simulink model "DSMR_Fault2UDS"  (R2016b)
settings: Solver=FixedStepDiscrete  StartTime=0.0  StopTime=10.0  FixedStep=0.02  RelTol=1e-3  EnableMultiTasking=on
undefined symbols (not defined in the file): bin2dec
libraries: simulink x312
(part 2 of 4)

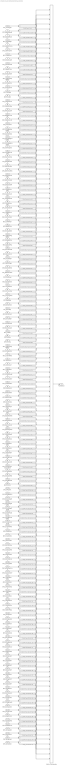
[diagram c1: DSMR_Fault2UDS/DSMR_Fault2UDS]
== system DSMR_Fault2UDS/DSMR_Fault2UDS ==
  DFC_CurrRngErr : Inport
  DFC_BattVoltRngErr : Inport  Port=2
  DFC_BattHVMsgTmt : Inport  Port=3
  DFC_BusHVMsgTmt : Inport  Port=4
  DFC_638LinCommErr : Inport  Port=5
  DFC_CellTempTmt : Inport  Port=6
  DFC_CellVoltTmt : Inport  Port=7
  DFC_InCanBusOff : Inport  Port=8
  DFC_VeCanBusOff : Inport  Port=9
  DFC_Msg2A3Tmt : Inport  Port=10
  DFC_RcMsg2A3Mis : Inport  Port=11
  DFC_ChkSumMsg2A3Err : Inport  Port=12
  DFC_RcMsg2A5Mis : Inport  Port=13
  DFC_RcMsg2A7Mis : Inport  Port=14
  DFC_CrashNpl : Inport  Port=15
  DFC_FuseNpl : Inport  Port=16
  DFC_Kl30cVoltLoErr : Inport  Port=17
  DFC_PosStuckMax : Inport  Port=18
  DFC_MPosStuckMin : Inport  Port=19
  DFC_MNegStuckMax : Inport  Port=20
  DFC_MNegStuckMin : Inport  Port=21
  DFC_PrStuckMin : Inport  Port=22
  DFC_DChrgPosStuckMax : Inport  Port=23
  DFC_DChrgPosStuckMin : Inport  Port=24
  DFC_DChrgNegStuckMax : Inport  Port=25
  DFC_DChrgNegStuckMin : Inport  Port=26
  DFC_HvPwrUpFail : Inport  Port=27
  DFC_DChrgPwrUpFail : Inport  Port=28
  DFC_BattTAlrmMax : Inport  Port=29
  DFC_BattTFaultMax : Inport  Port=30
  DFC_BattTAlrmMin : Inport  Port=31
  DFC_BattTFaultMin : Inport  Port=32
  DFC_BattTempVldMin : Inport  Port=33
  DFC_BattTCnstMax : Inport  Port=34
  DFC_BattTGradtMax : Inport  Port=35
  DFC_CellVoltAlrmMax : Inport  Port=36
  DFC_CellVoltFaultMax : Inport  Port=37
  DFC_CellVoltFusfMax : Inport  Port=38
  DFC_CellVoltAlrmMin : Inport  Port=39
  DFC_CellVoltFusfMin : Inport  Port=40
  DFC_CellVoltFaultMin : Inport  Port=41
  DFC_CellVoltVldMin : Inport  Port=42
  DFC_CellVoltNpl : Inport  Port=43
  DFC_Msg2E6Tmt : Inport  Port=44
  DFC_RcMsg2E6Mis : Inport  Port=45
  DFC_ChkSumMsg2E6Err : Inport  Port=46
  DFC_RcMsg2E1Mis : Inport  Port=47
  DFC_ChkSumMsg2E1Err : Inport  Port=48
  DFC_DcCanBusOff : Inport  Port=49
  DFC_DChrgTCnntMax : Inport  Port=50
  DFC_ChrgOCNpl : Inport  Port=51
  DFC_DisChOCNpl : Inport  Port=52
  DFC_BattVoltHiMax : Inport  Port=53
  DFC_BattVoltLoMin : Inport  Port=54
  DFC_ThmRnwy : Inport  Port=55
  DFC_AChrgPortOvrTemp : Inport  Port=56
  DFC_CurrOffsPlaus : Inport  Port=57
  DFC_CurrStukPlaus : Inport  Port=58
  DFC_CurrChrgPlaus : Inport  Port=59
  DFC_BattUNpl : Inport  Port=60
  DFC_BattVoltVld : Inport  Port=61
  DFC_PackUNpl : Inport  Port=62
  DFC_PackVoltVld : Inport  Port=63
  DFC_DChrgUNpl : Inport  Port=64
  DFC_DChrgVoltVld : Inport  Port=65
  DFC_BoardTempTmt : Inport  Port=66
  DFC_HvilMax : Inport  Port=67
  DFC_HvilMin : Inport  Port=68
  DFC_HvilSig : Inport  Port=69
  DFC_ChkSumMsg050Err : Inport  Port=70
  DFC_RcMsg050Mis : Inport  Port=71
  DFC_CrashHwNpl : Inport  Port=72
  DFC_IsoChkLv1 : Inport  Port=73
  DFC_IsoChkLv2 : Inport  Port=74
  DFC_InsResValdFault : Inport  Port=75
  DFC_Kl30OutRngErr : Inport  Port=76
  DFC_Kl30VoltLoErr : Inport  Port=77
  DFC_Kl30VoltHiErr : Inport  Port=78
  DFC_EepReadErr : Inport  Port=79
  DFC_BalStuckMax : Inport  Port=80
  DFC_BalStuckMin : Inport  Port=81
  DFC_CSCPwrSpyHiErr : Inport  Port=82
  DFC_CSCPwrSpyLoErr : Inport  Port=83
  DFC_CmcBordOTMax : Inport  Port=84
  DFC_BattTWarnMax : Inport  Port=85
  DFC_BattTWarnMin : Inport  Port=86
  DFC_BattTempVldMax : Inport  Port=87
  DFC_BattTHopMax : Inport  Port=88
  DFC_CellVoltRngHiErr : Inport  Port=89
  DFC_CellVoltRngLoErr : Inport  Port=90
  DFC_CellVoltWarnMax : Inport  Port=91
  DFC_CellVoltWarnMin : Inport  Port=92
  DFC_CellVoltVldMax : Inport  Port=93
  DFC_AChrgCurrMish : Inport  Port=94
  DFC_DChrgCurrMish : Inport  Port=95
  DFC_DChrgLowTempCurrMish : Inport  Port=96
  DFC_AChrgVoltMish : Inport  Port=97
  DFC_DChrgVoltMish : Inport  Port=98
  DFC_DChrgBattTMin : Inport  Port=99
  DFC_CC2Chk : Inport  Port=100
  DFC_APlusChk : Inport  Port=101
  DFC_DChrgMsgTmt : Inport  Port=102
  DFC_DChrgTNegElecMax : Inport  Port=103
  DFC_DChrgTNegElecMin : Inport  Port=104
  DFC_DChrgTNegElecSig : Inport  Port=105
  DFC_DChrgTPosElecMax : Inport  Port=106
  DFC_DChrgTPosElecMin : Inport  Port=107
  DFC_DChrgTPosElecSig : Inport  Port=108
  DFC_CcuSelfChkErr : Inport  Port=109
  DFC_ChrgOCMin : Inport  Port=110
  DFC_ChrgOCMax : Inport  Port=111
  DFC_DisChOCMin : Inport  Port=112
  DFC_DisChOCMax : Inport  Port=113
  DFC_SocRngLoMax : Inport  Port=114
  DFC_SocRngLoMin : Inport  Port=115
  DFC_SocRngHiMax : Inport  Port=116
  DFC_SocRngHiMin : Inport  Port=117
  DFC_InClntOverTmp : Inport  Port=118
  DFC_OutClntOverTmp : Inport  Port=119
  DFC_ClntDsTElecMax : Inport  Port=120
  DFC_ClntDsTElecMin : Inport  Port=121
  DFC_ClntDsTElecSig : Inport  Port=122
  DFC_ClntUsTElecMax : Inport  Port=123
  DFC_ClntUsTElecMin : Inport  Port=124
  DFC_ClntUsTElecSig : Inport  Port=125
  DFC_CoolPerfPlaus : Inport  Port=126
  DFC_HtgPerfPlaus : Inport  Port=127
  DFC_DChrgFobd : Inport  Port=128
  DFC_DChrgHvOnFail : Inport  Port=129
  DFC_AChgHVOnTmt : Inport  Port=130
  DFC_AChgHVOffTmt : Inport  Port=131
  DFC_AChgS2ClsdTmt : Inport  Port=132
  DFC_DChrgStakeErr : Inport  Port=133
  DFC_DChrgStkVoltErr : Inport  Port=134
  DFC_DChrgStkCurrErr : Inport  Port=135
  DFC_AChgPileRdyTmt : Inport  Port=136
  DFC_DChrgCHMTmt : Inport  Port=137
  DFC_DChrgCRMTmt : Inport  Port=138
  DFC_DChrgCMLTmt : Inport  Port=139
  DFC_DChrgCROTmt : Inport  Port=140
  DFC_DChrgCCSTmt : Inport  Port=141
  DFC_DChrgCSTTmt : Inport  Port=142
  DFC_DChrgCSDTmt : Inport  Port=143
  DFC_DChrgParaChk : Inport  Port=144
  DFC_DChrgCableChk : Inport  Port=145
  DFC_DChrgSLACTOut : Inport  Port=146
  DFC_DChrgCnntErr : Inport  Port=147
  DFC_DChrgLckErr : Inport  Port=148
  DFC_AChrgCnntErr : Inport  Port=149
  DFC_AChgLckTmt : Inport  Port=150
  DFC_AChgRdyPndiTmt : Inport  Port=151
  DFC_AChgRdyTmt : Inport  Port=152
  DFC_AChgingErr : Inport  Port=153
  DFC_AChgUnlckTmt : Inport  Port=154
  DFC_AChgFobd : Inport  Port=155
  DFC_SocValJmp : Inport  Port=156
  DSM_GetSFCErD : Subsystem  TreatAsAtomicUnit=on  RTWFcnName=TONV_10msTimeDebounce  RTWFileName=SrvLib
  DSM_GetSFCErD1 : Subsystem  TreatAsAtomicUnit=on  RTWFcnName=TONV_10msTimeDebounce  RTWFileName=SrvLib
  DSM_GetSFCErD10 : Subsystem  TreatAsAtomicUnit=on  RTWFcnName=TONV_10msTimeDebounce  RTWFileName=SrvLib
  DSM_GetSFCErD100 : Subsystem  TreatAsAtomicUnit=on  RTWFcnName=TONV_10msTimeDebounce  RTWFileName=SrvLib
  DSM_GetSFCErD101 : Subsystem  TreatAsAtomicUnit=on  RTWFcnName=TONV_10msTimeDebounce  RTWFileName=SrvLib
  DSM_GetSFCErD102 : Subsystem  TreatAsAtomicUnit=on  RTWFcnName=TONV_10msTimeDebounce  RTWFileName=SrvLib
  DSM_GetSFCErD103 : Subsystem  TreatAsAtomicUnit=on  RTWFcnName=TONV_10msTimeDebounce  RTWFileName=SrvLib
  DSM_GetSFCErD104 : Subsystem  TreatAsAtomicUnit=on  RTWFcnName=TONV_10msTimeDebounce  RTWFileName=SrvLib
  DSM_GetSFCErD105 : Subsystem  TreatAsAtomicUnit=on  RTWFcnName=TONV_10msTimeDebounce  RTWFileName=SrvLib
  DSM_GetSFCErD106 : Subsystem  TreatAsAtomicUnit=on  RTWFcnName=TONV_10msTimeDebounce  RTWFileName=SrvLib
  DSM_GetSFCErD107 : Subsystem  TreatAsAtomicUnit=on  RTWFcnName=TONV_10msTimeDebounce  RTWFileName=SrvLib
  DSM_GetSFCErD108 : Subsystem  TreatAsAtomicUnit=on  RTWFcnName=TONV_10msTimeDebounce  RTWFileName=SrvLib
  DSM_GetSFCErD109 : Subsystem  TreatAsAtomicUnit=on  RTWFcnName=TONV_10msTimeDebounce  RTWFileName=SrvLib
  DSM_GetSFCErD11 : Subsystem  TreatAsAtomicUnit=on  RTWFcnName=TONV_10msTimeDebounce  RTWFileName=SrvLib
  DSM_GetSFCErD110 : Subsystem  TreatAsAtomicUnit=on  RTWFcnName=TONV_10msTimeDebounce  RTWFileName=SrvLib
  DSM_GetSFCErD111 : Subsystem  TreatAsAtomicUnit=on  RTWFcnName=TONV_10msTimeDebounce  RTWFileName=SrvLib
  DSM_GetSFCErD112 : Subsystem  TreatAsAtomicUnit=on  RTWFcnName=TONV_10msTimeDebounce  RTWFileName=SrvLib
  DSM_GetSFCErD113 : Subsystem  TreatAsAtomicUnit=on  RTWFcnName=TONV_10msTimeDebounce  RTWFileName=SrvLib
  DSM_GetSFCErD114 : Subsystem  TreatAsAtomicUnit=on  RTWFcnName=TONV_10msTimeDebounce  RTWFileName=SrvLib
  DSM_GetSFCErD115 : Subsystem  TreatAsAtomicUnit=on  RTWFcnName=TONV_10msTimeDebounce  RTWFileName=SrvLib
  DSM_GetSFCErD116 : Subsystem  TreatAsAtomicUnit=on  RTWFcnName=TONV_10msTimeDebounce  RTWFileName=SrvLib
  DSM_GetSFCErD117 : Subsystem  TreatAsAtomicUnit=on  RTWFcnName=TONV_10msTimeDebounce  RTWFileName=SrvLib
  DSM_GetSFCErD118 : Subsystem  TreatAsAtomicUnit=on  RTWFcnName=TONV_10msTimeDebounce  RTWFileName=SrvLib
  DSM_GetSFCErD119 : Subsystem  TreatAsAtomicUnit=on  RTWFcnName=TONV_10msTimeDebounce  RTWFileName=SrvLib
  DSM_GetSFCErD12 : Subsystem  TreatAsAtomicUnit=on  RTWFcnName=TONV_10msTimeDebounce  RTWFileName=SrvLib
  DSM_GetSFCErD120 : Subsystem  TreatAsAtomicUnit=on  RTWFcnName=TONV_10msTimeDebounce  RTWFileName=SrvLib
  DSM_GetSFCErD121 : Subsystem  TreatAsAtomicUnit=on  RTWFcnName=TONV_10msTimeDebounce  RTWFileName=SrvLib
  DSM_GetSFCErD122 : Subsystem  TreatAsAtomicUnit=on  RTWFcnName=TONV_10msTimeDebounce  RTWFileName=SrvLib
  DSM_GetSFCErD123 : Subsystem  TreatAsAtomicUnit=on  RTWFcnName=TONV_10msTimeDebounce  RTWFileName=SrvLib
  DSM_GetSFCErD124 : Subsystem  TreatAsAtomicUnit=on  RTWFcnName=TONV_10msTimeDebounce  RTWFileName=SrvLib
  DSM_GetSFCErD125 : Subsystem  TreatAsAtomicUnit=on  RTWFcnName=TONV_10msTimeDebounce  RTWFileName=SrvLib
  DSM_GetSFCErD126 : Subsystem  TreatAsAtomicUnit=on  RTWFcnName=TONV_10msTimeDebounce  RTWFileName=SrvLib
  DSM_GetSFCErD127 : Subsystem  TreatAsAtomicUnit=on  RTWFcnName=TONV_10msTimeDebounce  RTWFileName=SrvLib
  DSM_GetSFCErD128 : Subsystem  TreatAsAtomicUnit=on  RTWFcnName=TONV_10msTimeDebounce  RTWFileName=SrvLib
  DSM_GetSFCErD129 : Subsystem  TreatAsAtomicUnit=on  RTWFcnName=TONV_10msTimeDebounce  RTWFileName=SrvLib
  DSM_GetSFCErD13 : Subsystem  TreatAsAtomicUnit=on  RTWFcnName=TONV_10msTimeDebounce  RTWFileName=SrvLib
  DSM_GetSFCErD130 : Subsystem  TreatAsAtomicUnit=on  RTWFcnName=TONV_10msTimeDebounce  RTWFileName=SrvLib
  DSM_GetSFCErD131 : Subsystem  TreatAsAtomicUnit=on  RTWFcnName=TONV_10msTimeDebounce  RTWFileName=SrvLib
  DSM_GetSFCErD132 : Subsystem  TreatAsAtomicUnit=on  RTWFcnName=TONV_10msTimeDebounce  RTWFileName=SrvLib
  DSM_GetSFCErD133 : Subsystem  TreatAsAtomicUnit=on  RTWFcnName=TONV_10msTimeDebounce  RTWFileName=SrvLib
  DSM_GetSFCErD134 : Subsystem  TreatAsAtomicUnit=on  RTWFcnName=TONV_10msTimeDebounce  RTWFileName=SrvLib
  DSM_GetSFCErD135 : Subsystem  TreatAsAtomicUnit=on  RTWFcnName=TONV_10msTimeDebounce  RTWFileName=SrvLib
  DSM_GetSFCErD136 : Subsystem  TreatAsAtomicUnit=on  RTWFcnName=TONV_10msTimeDebounce  RTWFileName=SrvLib
  DSM_GetSFCErD137 : Subsystem  TreatAsAtomicUnit=on  RTWFcnName=TONV_10msTimeDebounce  RTWFileName=SrvLib
  DSM_GetSFCErD138 : Subsystem  TreatAsAtomicUnit=on  RTWFcnName=TONV_10msTimeDebounce  RTWFileName=SrvLib
  DSM_GetSFCErD139 : Subsystem  TreatAsAtomicUnit=on  RTWFcnName=TONV_10msTimeDebounce  RTWFileName=SrvLib
  DSM_GetSFCErD14 : Subsystem  TreatAsAtomicUnit=on  RTWFcnName=TONV_10msTimeDebounce  RTWFileName=SrvLib
  DSM_GetSFCErD140 : Subsystem  TreatAsAtomicUnit=on  RTWFcnName=TONV_10msTimeDebounce  RTWFileName=SrvLib
  DSM_GetSFCErD141 : Subsystem  TreatAsAtomicUnit=on  RTWFcnName=TONV_10msTimeDebounce  RTWFileName=SrvLib
  DSM_GetSFCErD142 : Subsystem  TreatAsAtomicUnit=on  RTWFcnName=TONV_10msTimeDebounce  RTWFileName=SrvLib
  DSM_GetSFCErD143 : Subsystem  TreatAsAtomicUnit=on  RTWFcnName=TONV_10msTimeDebounce  RTWFileName=SrvLib
  DSM_GetSFCErD144 : Subsystem  TreatAsAtomicUnit=on  RTWFcnName=TONV_10msTimeDebounce  RTWFileName=SrvLib
  DSM_GetSFCErD145 : Subsystem  TreatAsAtomicUnit=on  RTWFcnName=TONV_10msTimeDebounce  RTWFileName=SrvLib
  DSM_GetSFCErD146 : Subsystem  TreatAsAtomicUnit=on  RTWFcnName=TONV_10msTimeDebounce  RTWFileName=SrvLib
  DSM_GetSFCErD147 : Subsystem  TreatAsAtomicUnit=on  RTWFcnName=TONV_10msTimeDebounce  RTWFileName=SrvLib
  DSM_GetSFCErD148 : Subsystem  TreatAsAtomicUnit=on  RTWFcnName=TONV_10msTimeDebounce  RTWFileName=SrvLib
  DSM_GetSFCErD149 : Subsystem  TreatAsAtomicUnit=on  RTWFcnName=TONV_10msTimeDebounce  RTWFileName=SrvLib
  DSM_GetSFCErD15 : Subsystem  TreatAsAtomicUnit=on  RTWFcnName=TONV_10msTimeDebounce  RTWFileName=SrvLib
  DSM_GetSFCErD150 : Subsystem  TreatAsAtomicUnit=on  RTWFcnName=TONV_10msTimeDebounce  RTWFileName=SrvLib
  DSM_GetSFCErD151 : Subsystem  TreatAsAtomicUnit=on  RTWFcnName=TONV_10msTimeDebounce  RTWFileName=SrvLib
  DSM_GetSFCErD152 : Subsystem  TreatAsAtomicUnit=on  RTWFcnName=TONV_10msTimeDebounce  RTWFileName=SrvLib
  DSM_GetSFCErD153 : Subsystem  TreatAsAtomicUnit=on  RTWFcnName=TONV_10msTimeDebounce  RTWFileName=SrvLib
  DSM_GetSFCErD154 : Subsystem  TreatAsAtomicUnit=on  RTWFcnName=TONV_10msTimeDebounce  RTWFileName=SrvLib
  DSM_GetSFCErD155 : Subsystem  TreatAsAtomicUnit=on  RTWFcnName=TONV_10msTimeDebounce  RTWFileName=SrvLib
  DSM_GetSFCErD16 : Subsystem  TreatAsAtomicUnit=on  RTWFcnName=TONV_10msTimeDebounce  RTWFileName=SrvLib
  DSM_GetSFCErD17 : Subsystem  TreatAsAtomicUnit=on  RTWFcnName=TONV_10msTimeDebounce  RTWFileName=SrvLib
  DSM_GetSFCErD18 : Subsystem  TreatAsAtomicUnit=on  RTWFcnName=TONV_10msTimeDebounce  RTWFileName=SrvLib
  DSM_GetSFCErD19 : Subsystem  TreatAsAtomicUnit=on  RTWFcnName=TONV_10msTimeDebounce  RTWFileName=SrvLib
  DSM_GetSFCErD2 : Subsystem  TreatAsAtomicUnit=on  RTWFcnName=TONV_10msTimeDebounce  RTWFileName=SrvLib
  DSM_GetSFCErD20 : Subsystem  TreatAsAtomicUnit=on  RTWFcnName=TONV_10msTimeDebounce  RTWFileName=SrvLib
  DSM_GetSFCErD21 : Subsystem  TreatAsAtomicUnit=on  RTWFcnName=TONV_10msTimeDebounce  RTWFileName=SrvLib
  DSM_GetSFCErD22 : Subsystem  TreatAsAtomicUnit=on  RTWFcnName=TONV_10msTimeDebounce  RTWFileName=SrvLib
  DSM_GetSFCErD23 : Subsystem  TreatAsAtomicUnit=on  RTWFcnName=TONV_10msTimeDebounce  RTWFileName=SrvLib
  DSM_GetSFCErD24 : Subsystem  TreatAsAtomicUnit=on  RTWFcnName=TONV_10msTimeDebounce  RTWFileName=SrvLib
  DSM_GetSFCErD25 : Subsystem  TreatAsAtomicUnit=on  RTWFcnName=TONV_10msTimeDebounce  RTWFileName=SrvLib
  DSM_GetSFCErD26 : Subsystem  TreatAsAtomicUnit=on  RTWFcnName=TONV_10msTimeDebounce  RTWFileName=SrvLib
  DSM_GetSFCErD27 : Subsystem  TreatAsAtomicUnit=on  RTWFcnName=TONV_10msTimeDebounce  RTWFileName=SrvLib
  DSM_GetSFCErD28 : Subsystem  TreatAsAtomicUnit=on  RTWFcnName=TONV_10msTimeDebounce  RTWFileName=SrvLib
  DSM_GetSFCErD29 : Subsystem  TreatAsAtomicUnit=on  RTWFcnName=TONV_10msTimeDebounce  RTWFileName=SrvLib
  DSM_GetSFCErD3 : Subsystem  TreatAsAtomicUnit=on  RTWFcnName=TONV_10msTimeDebounce  RTWFileName=SrvLib
  DSM_GetSFCErD30 : Subsystem  TreatAsAtomicUnit=on  RTWFcnName=TONV_10msTimeDebounce  RTWFileName=SrvLib
  DSM_GetSFCErD31 : Subsystem  TreatAsAtomicUnit=on  RTWFcnName=TONV_10msTimeDebounce  RTWFileName=SrvLib
  DSM_GetSFCErD32 : Subsystem  TreatAsAtomicUnit=on  RTWFcnName=TONV_10msTimeDebounce  RTWFileName=SrvLib
  DSM_GetSFCErD33 : Subsystem  TreatAsAtomicUnit=on  RTWFcnName=TONV_10msTimeDebounce  RTWFileName=SrvLib
  DSM_GetSFCErD34 : Subsystem  TreatAsAtomicUnit=on  RTWFcnName=TONV_10msTimeDebounce  RTWFileName=SrvLib
  DSM_GetSFCErD35 : Subsystem  TreatAsAtomicUnit=on  RTWFcnName=TONV_10msTimeDebounce  RTWFileName=SrvLib
  DSM_GetSFCErD36 : Subsystem  TreatAsAtomicUnit=on  RTWFcnName=TONV_10msTimeDebounce  RTWFileName=SrvLib
  DSM_GetSFCErD37 : Subsystem  TreatAsAtomicUnit=on  RTWFcnName=TONV_10msTimeDebounce  RTWFileName=SrvLib
  DSM_GetSFCErD38 : Subsystem  TreatAsAtomicUnit=on  RTWFcnName=TONV_10msTimeDebounce  RTWFileName=SrvLib
  DSM_GetSFCErD39 : Subsystem  TreatAsAtomicUnit=on  RTWFcnName=TONV_10msTimeDebounce  RTWFileName=SrvLib
  DSM_GetSFCErD4 : Subsystem  TreatAsAtomicUnit=on  RTWFcnName=TONV_10msTimeDebounce  RTWFileName=SrvLib
  DSM_GetSFCErD40 : Subsystem  TreatAsAtomicUnit=on  RTWFcnName=TONV_10msTimeDebounce  RTWFileName=SrvLib
  DSM_GetSFCErD41 : Subsystem  TreatAsAtomicUnit=on  RTWFcnName=TONV_10msTimeDebounce  RTWFileName=SrvLib
  DSM_GetSFCErD42 : Subsystem  TreatAsAtomicUnit=on  RTWFcnName=TONV_10msTimeDebounce  RTWFileName=SrvLib
  DSM_GetSFCErD43 : Subsystem  TreatAsAtomicUnit=on  RTWFcnName=TONV_10msTimeDebounce  RTWFileName=SrvLib
  DSM_GetSFCErD44 : Subsystem  TreatAsAtomicUnit=on  RTWFcnName=TONV_10msTimeDebounce  RTWFileName=SrvLib
  DSM_GetSFCErD45 : Subsystem  TreatAsAtomicUnit=on  RTWFcnName=TONV_10msTimeDebounce  RTWFileName=SrvLib
  DSM_GetSFCErD46 : Subsystem  TreatAsAtomicUnit=on  RTWFcnName=TONV_10msTimeDebounce  RTWFileName=SrvLib
  DSM_GetSFCErD47 : Subsystem  TreatAsAtomicUnit=on  RTWFcnName=TONV_10msTimeDebounce  RTWFileName=SrvLib
  DSM_GetSFCErD48 : Subsystem  TreatAsAtomicUnit=on  RTWFcnName=TONV_10msTimeDebounce  RTWFileName=SrvLib
  DSM_GetSFCErD49 : Subsystem  TreatAsAtomicUnit=on  RTWFcnName=TONV_10msTimeDebounce  RTWFileName=SrvLib
  DSM_GetSFCErD5 : Subsystem  TreatAsAtomicUnit=on  RTWFcnName=TONV_10msTimeDebounce  RTWFileName=SrvLib
  DSM_GetSFCErD50 : Subsystem  TreatAsAtomicUnit=on  RTWFcnName=TONV_10msTimeDebounce  RTWFileName=SrvLib
  DSM_GetSFCErD51 : Subsystem  TreatAsAtomicUnit=on  RTWFcnName=TONV_10msTimeDebounce  RTWFileName=SrvLib
  DSM_GetSFCErD52 : Subsystem  TreatAsAtomicUnit=on  RTWFcnName=TONV_10msTimeDebounce  RTWFileName=SrvLib
  DSM_GetSFCErD53 : Subsystem  TreatAsAtomicUnit=on  RTWFcnName=TONV_10msTimeDebounce  RTWFileName=SrvLib
  DSM_GetSFCErD54 : Subsystem  TreatAsAtomicUnit=on  RTWFcnName=TONV_10msTimeDebounce  RTWFileName=SrvLib
  DSM_GetSFCErD55 : Subsystem  TreatAsAtomicUnit=on  RTWFcnName=TONV_10msTimeDebounce  RTWFileName=SrvLib
  DSM_GetSFCErD56 : Subsystem  TreatAsAtomicUnit=on  RTWFcnName=TONV_10msTimeDebounce  RTWFileName=SrvLib
  DSM_GetSFCErD57 : Subsystem  TreatAsAtomicUnit=on  RTWFcnName=TONV_10msTimeDebounce  RTWFileName=SrvLib
  DSM_GetSFCErD58 : Subsystem  TreatAsAtomicUnit=on  RTWFcnName=TONV_10msTimeDebounce  RTWFileName=SrvLib
  DSM_GetSFCErD59 : Subsystem  TreatAsAtomicUnit=on  RTWFcnName=TONV_10msTimeDebounce  RTWFileName=SrvLib
  DSM_GetSFCErD6 : Subsystem  TreatAsAtomicUnit=on  RTWFcnName=TONV_10msTimeDebounce  RTWFileName=SrvLib
  DSM_GetSFCErD60 : Subsystem  TreatAsAtomicUnit=on  RTWFcnName=TONV_10msTimeDebounce  RTWFileName=SrvLib
  DSM_GetSFCErD61 : Subsystem  TreatAsAtomicUnit=on  RTWFcnName=TONV_10msTimeDebounce  RTWFileName=SrvLib
  DSM_GetSFCErD62 : Subsystem  TreatAsAtomicUnit=on  RTWFcnName=TONV_10msTimeDebounce  RTWFileName=SrvLib
  DSM_GetSFCErD63 : Subsystem  TreatAsAtomicUnit=on  RTWFcnName=TONV_10msTimeDebounce  RTWFileName=SrvLib
  DSM_GetSFCErD64 : Subsystem  TreatAsAtomicUnit=on  RTWFcnName=TONV_10msTimeDebounce  RTWFileName=SrvLib
  DSM_GetSFCErD65 : Subsystem  TreatAsAtomicUnit=on  RTWFcnName=TONV_10msTimeDebounce  RTWFileName=SrvLib
  DSM_GetSFCErD66 : Subsystem  TreatAsAtomicUnit=on  RTWFcnName=TONV_10msTimeDebounce  RTWFileName=SrvLib
  DSM_GetSFCErD67 : Subsystem  TreatAsAtomicUnit=on  RTWFcnName=TONV_10msTimeDebounce  RTWFileName=SrvLib
  DSM_GetSFCErD68 : Subsystem  TreatAsAtomicUnit=on  RTWFcnName=TONV_10msTimeDebounce  RTWFileName=SrvLib
  DSM_GetSFCErD69 : Subsystem  TreatAsAtomicUnit=on  RTWFcnName=TONV_10msTimeDebounce  RTWFileName=SrvLib
  DSM_GetSFCErD7 : Subsystem  TreatAsAtomicUnit=on  RTWFcnName=TONV_10msTimeDebounce  RTWFileName=SrvLib
  DSM_GetSFCErD70 : Subsystem  TreatAsAtomicUnit=on  RTWFcnName=TONV_10msTimeDebounce  RTWFileName=SrvLib
  DSM_GetSFCErD71 : Subsystem  TreatAsAtomicUnit=on  RTWFcnName=TONV_10msTimeDebounce  RTWFileName=SrvLib
  DSM_GetSFCErD72 : Subsystem  TreatAsAtomicUnit=on  RTWFcnName=TONV_10msTimeDebounce  RTWFileName=SrvLib
  DSM_GetSFCErD73 : Subsystem  TreatAsAtomicUnit=on  RTWFcnName=TONV_10msTimeDebounce  RTWFileName=SrvLib
  DSM_GetSFCErD74 : Subsystem  TreatAsAtomicUnit=on  RTWFcnName=TONV_10msTimeDebounce  RTWFileName=SrvLib
  DSM_GetSFCErD75 : Subsystem  TreatAsAtomicUnit=on  RTWFcnName=TONV_10msTimeDebounce  RTWFileName=SrvLib
  DSM_GetSFCErD76 : Subsystem  TreatAsAtomicUnit=on  RTWFcnName=TONV_10msTimeDebounce  RTWFileName=SrvLib
  DSM_GetSFCErD77 : Subsystem  TreatAsAtomicUnit=on  RTWFcnName=TONV_10msTimeDebounce  RTWFileName=SrvLib
  DSM_GetSFCErD78 : Subsystem  TreatAsAtomicUnit=on  RTWFcnName=TONV_10msTimeDebounce  RTWFileName=SrvLib
  DSM_GetSFCErD79 : Subsystem  TreatAsAtomicUnit=on  RTWFcnName=TONV_10msTimeDebounce  RTWFileName=SrvLib
  DSM_GetSFCErD8 : Subsystem  TreatAsAtomicUnit=on  RTWFcnName=TONV_10msTimeDebounce  RTWFileName=SrvLib
  DSM_GetSFCErD80 : Subsystem  TreatAsAtomicUnit=on  RTWFcnName=TONV_10msTimeDebounce  RTWFileName=SrvLib
  DSM_GetSFCErD81 : Subsystem  TreatAsAtomicUnit=on  RTWFcnName=TONV_10msTimeDebounce  RTWFileName=SrvLib
  DSM_GetSFCErD82 : Subsystem  TreatAsAtomicUnit=on  RTWFcnName=TONV_10msTimeDebounce  RTWFileName=SrvLib
  DSM_GetSFCErD83 : Subsystem  TreatAsAtomicUnit=on  RTWFcnName=TONV_10msTimeDebounce  RTWFileName=SrvLib
  DSM_GetSFCErD84 : Subsystem  TreatAsAtomicUnit=on  RTWFcnName=TONV_10msTimeDebounce  RTWFileName=SrvLib
  DSM_GetSFCErD85 : Subsystem  TreatAsAtomicUnit=on  RTWFcnName=TONV_10msTimeDebounce  RTWFileName=SrvLib
  DSM_GetSFCErD86 : Subsystem  TreatAsAtomicUnit=on  RTWFcnName=TONV_10msTimeDebounce  RTWFileName=SrvLib
  DSM_GetSFCErD87 : Subsystem  TreatAsAtomicUnit=on  RTWFcnName=TONV_10msTimeDebounce  RTWFileName=SrvLib
  DSM_GetSFCErD88 : Subsystem  TreatAsAtomicUnit=on  RTWFcnName=TONV_10msTimeDebounce  RTWFileName=SrvLib
  DSM_GetSFCErD89 : Subsystem  TreatAsAtomicUnit=on  RTWFcnName=TONV_10msTimeDebounce  RTWFileName=SrvLib
  DSM_GetSFCErD9 : Subsystem  TreatAsAtomicUnit=on  RTWFcnName=TONV_10msTimeDebounce  RTWFileName=SrvLib
  DSM_GetSFCErD90 : Subsystem  TreatAsAtomicUnit=on  RTWFcnName=TONV_10msTimeDebounce  RTWFileName=SrvLib
  DSM_GetSFCErD91 : Subsystem  TreatAsAtomicUnit=on  RTWFcnName=TONV_10msTimeDebounce  RTWFileName=SrvLib
  DSM_GetSFCErD92 : Subsystem  TreatAsAtomicUnit=on  RTWFcnName=TONV_10msTimeDebounce  RTWFileName=SrvLib
  DSM_GetSFCErD93 : Subsystem  TreatAsAtomicUnit=on  RTWFcnName=TONV_10msTimeDebounce  RTWFileName=SrvLib
  DSM_GetSFCErD94 : Subsystem  TreatAsAtomicUnit=on  RTWFcnName=TONV_10msTimeDebounce  RTWFileName=SrvLib
  DSM_GetSFCErD95 : Subsystem  TreatAsAtomicUnit=on  RTWFcnName=TONV_10msTimeDebounce  RTWFileName=SrvLib
  DSM_GetSFCErD96 : Subsystem  TreatAsAtomicUnit=on  RTWFcnName=TONV_10msTimeDebounce  RTWFileName=SrvLib
  DSM_GetSFCErD97 : Subsystem  TreatAsAtomicUnit=on  RTWFcnName=TONV_10msTimeDebounce  RTWFileName=SrvLib
  DSM_GetSFCErD98 : Subsystem  TreatAsAtomicUnit=on  RTWFcnName=TONV_10msTimeDebounce  RTWFileName=SrvLib
  DSM_GetSFCErD99 : Subsystem  TreatAsAtomicUnit=on  RTWFcnName=TONV_10msTimeDebounce  RTWFileName=SrvLib
  Vector Concatenate : Concatenate  NumInputs=156
  FaultStatus : Outport
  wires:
  DFC_CurrRngErr/1 -> DSM_GetSFCErD/1(DFC)
  DFC_BattVoltRngErr/1 -> DSM_GetSFCErD1/1(DFC)
  DFC_BattHVMsgTmt/1 -> DSM_GetSFCErD2/1(DFC)
  DFC_BusHVMsgTmt/1 -> DSM_GetSFCErD3/1(DFC)
  DFC_638LinCommErr/1 -> DSM_GetSFCErD4/1(DFC)
  DFC_CellTempTmt/1 -> DSM_GetSFCErD5/1(DFC)
  DFC_CellVoltTmt/1 -> DSM_GetSFCErD6/1(DFC)
  DFC_InCanBusOff/1 -> DSM_GetSFCErD7/1(DFC)
  DFC_VeCanBusOff/1 -> DSM_GetSFCErD8/1(DFC)
  DFC_Msg2A3Tmt/1 -> DSM_GetSFCErD9/1(DFC)
  DFC_RcMsg2A3Mis/1 -> DSM_GetSFCErD10/1(DFC)
  DFC_ChkSumMsg2A3Err/1 -> DSM_GetSFCErD11/1(DFC)
  DFC_RcMsg2A5Mis/1 -> DSM_GetSFCErD12/1(DFC)
  DFC_RcMsg2A7Mis/1 -> DSM_GetSFCErD13/1(DFC)
  DFC_CrashNpl/1 -> DSM_GetSFCErD14/1(DFC)
  DFC_FuseNpl/1 -> DSM_GetSFCErD15/1(DFC)
  DFC_Kl30cVoltLoErr/1 -> DSM_GetSFCErD16/1(DFC)
  DFC_PosStuckMax/1 -> DSM_GetSFCErD17/1(DFC)
  DFC_MPosStuckMin/1 -> DSM_GetSFCErD18/1(DFC)
  DFC_MNegStuckMax/1 -> DSM_GetSFCErD19/1(DFC)
  DFC_MNegStuckMin/1 -> DSM_GetSFCErD20/1(DFC)
  DFC_PrStuckMin/1 -> DSM_GetSFCErD21/1(DFC)
  DFC_DChrgPosStuckMax/1 -> DSM_GetSFCErD22/1(DFC)
  DFC_DChrgPosStuckMin/1 -> DSM_GetSFCErD23/1(DFC)
  DFC_DChrgNegStuckMax/1 -> DSM_GetSFCErD24/1(DFC)
  DFC_DChrgNegStuckMin/1 -> DSM_GetSFCErD25/1(DFC)
  DFC_HvPwrUpFail/1 -> DSM_GetSFCErD26/1(DFC)
  DFC_DChrgPwrUpFail/1 -> DSM_GetSFCErD27/1(DFC)
  DFC_BattTAlrmMax/1 -> DSM_GetSFCErD28/1(DFC)
  DFC_BattTFaultMax/1 -> DSM_GetSFCErD29/1(DFC)
  DFC_BattTAlrmMin/1 -> DSM_GetSFCErD30/1(DFC)
  DFC_BattTFaultMin/1 -> DSM_GetSFCErD31/1(DFC)
  DFC_BattTempVldMin/1 -> DSM_GetSFCErD32/1(DFC)
  DFC_BattTCnstMax/1 -> DSM_GetSFCErD33/1(DFC)
  DFC_BattTGradtMax/1 -> DSM_GetSFCErD34/1(DFC)
  DFC_CellVoltAlrmMax/1 -> DSM_GetSFCErD35/1(DFC)
  DFC_CellVoltFaultMax/1 -> DSM_GetSFCErD36/1(DFC)
  DFC_CellVoltFusfMax/1 -> DSM_GetSFCErD37/1(DFC)
  DFC_CellVoltAlrmMin/1 -> DSM_GetSFCErD38/1(DFC)
  DFC_CellVoltFusfMin/1 -> DSM_GetSFCErD39/1(DFC)
  DFC_CellVoltFaultMin/1 -> DSM_GetSFCErD40/1(DFC)
  DFC_CellVoltVldMin/1 -> DSM_GetSFCErD41/1(DFC)
  DFC_CellVoltNpl/1 -> DSM_GetSFCErD42/1(DFC)
  DFC_Msg2E6Tmt/1 -> DSM_GetSFCErD43/1(DFC)
  DFC_RcMsg2E6Mis/1 -> DSM_GetSFCErD44/1(DFC)
  DFC_ChkSumMsg2E6Err/1 -> DSM_GetSFCErD45/1(DFC)
  DFC_RcMsg2E1Mis/1 -> DSM_GetSFCErD46/1(DFC)
  DFC_ChkSumMsg2E1Err/1 -> DSM_GetSFCErD47/1(DFC)
  DFC_DcCanBusOff/1 -> DSM_GetSFCErD48/1(DFC)
  DFC_DChrgTCnntMax/1 -> DSM_GetSFCErD49/1(DFC)
  DFC_ChrgOCNpl/1 -> DSM_GetSFCErD50/1(DFC)
  DFC_DisChOCNpl/1 -> DSM_GetSFCErD51/1(DFC)
  DFC_BattVoltHiMax/1 -> DSM_GetSFCErD52/1(DFC)
  DFC_BattVoltLoMin/1 -> DSM_GetSFCErD53/1(DFC)
  DFC_ThmRnwy/1 -> DSM_GetSFCErD54/1(DFC)
  DFC_AChrgPortOvrTemp/1 -> DSM_GetSFCErD55/1(DFC)
  DFC_CurrOffsPlaus/1 -> DSM_GetSFCErD56/1(DFC)
  DFC_CurrStukPlaus/1 -> DSM_GetSFCErD57/1(DFC)
  DFC_CurrChrgPlaus/1 -> DSM_GetSFCErD58/1(DFC)
  DFC_BattUNpl/1 -> DSM_GetSFCErD59/1(DFC)
  DFC_BattVoltVld/1 -> DSM_GetSFCErD60/1(DFC)
  DFC_PackUNpl/1 -> DSM_GetSFCErD61/1(DFC)
  DFC_PackVoltVld/1 -> DSM_GetSFCErD62/1(DFC)
  DFC_DChrgUNpl/1 -> DSM_GetSFCErD63/1(DFC)
  DFC_DChrgVoltVld/1 -> DSM_GetSFCErD64/1(DFC)
  DFC_BoardTempTmt/1 -> DSM_GetSFCErD65/1(DFC)
  DFC_HvilMax/1 -> DSM_GetSFCErD66/1(DFC)
  DFC_HvilMin/1 -> DSM_GetSFCErD67/1(DFC)
  DFC_HvilSig/1 -> DSM_GetSFCErD68/1(DFC)
  DFC_ChkSumMsg050Err/1 -> DSM_GetSFCErD69/1(DFC)
  DFC_RcMsg050Mis/1 -> DSM_GetSFCErD70/1(DFC)
  DFC_CrashHwNpl/1 -> DSM_GetSFCErD71/1(DFC)
  DFC_IsoChkLv1/1 -> DSM_GetSFCErD72/1(DFC)
  DFC_IsoChkLv2/1 -> DSM_GetSFCErD73/1(DFC)
  DFC_InsResValdFault/1 -> DSM_GetSFCErD74/1(DFC)
  DFC_Kl30OutRngErr/1 -> DSM_GetSFCErD75/1(DFC)
  DFC_Kl30VoltLoErr/1 -> DSM_GetSFCErD76/1(DFC)
  DFC_Kl30VoltHiErr/1 -> DSM_GetSFCErD77/1(DFC)
  DFC_EepReadErr/1 -> DSM_GetSFCErD78/1(DFC)
  DFC_BalStuckMax/1 -> DSM_GetSFCErD79/1(DFC)
  DFC_BalStuckMin/1 -> DSM_GetSFCErD80/1(DFC)
  DFC_CSCPwrSpyHiErr/1 -> DSM_GetSFCErD81/1(DFC)
  DFC_CSCPwrSpyLoErr/1 -> DSM_GetSFCErD82/1(DFC)
  DFC_CmcBordOTMax/1 -> DSM_GetSFCErD83/1(DFC)
  DFC_BattTWarnMax/1 -> DSM_GetSFCErD84/1(DFC)
  DFC_BattTWarnMin/1 -> DSM_GetSFCErD85/1(DFC)
  DFC_BattTempVldMax/1 -> DSM_GetSFCErD86/1(DFC)
  DFC_BattTHopMax/1 -> DSM_GetSFCErD87/1(DFC)
  DFC_CellVoltRngHiErr/1 -> DSM_GetSFCErD88/1(DFC)
  DFC_CellVoltRngLoErr/1 -> DSM_GetSFCErD89/1(DFC)
  DFC_CellVoltWarnMax/1 -> DSM_GetSFCErD90/1(DFC)
  DFC_CellVoltWarnMin/1 -> DSM_GetSFCErD91/1(DFC)
  DFC_CellVoltVldMax/1 -> DSM_GetSFCErD92/1(DFC)
  DFC_AChrgCurrMish/1 -> DSM_GetSFCErD93/1(DFC)
  DFC_DChrgCurrMish/1 -> DSM_GetSFCErD94/1(DFC)
  DFC_DChrgLowTempCurrMish/1 -> DSM_GetSFCErD95/1(DFC)
  DFC_AChrgVoltMish/1 -> DSM_GetSFCErD96/1(DFC)
  DFC_DChrgVoltMish/1 -> DSM_GetSFCErD97/1(DFC)
  DFC_DChrgBattTMin/1 -> DSM_GetSFCErD98/1(DFC)
  DFC_CC2Chk/1 -> DSM_GetSFCErD99/1(DFC)
  DFC_APlusChk/1 -> DSM_GetSFCErD100/1(DFC)
  DFC_DChrgMsgTmt/1 -> DSM_GetSFCErD101/1(DFC)
  DFC_DChrgTNegElecMax/1 -> DSM_GetSFCErD102/1(DFC)
  DFC_DChrgTNegElecMin/1 -> DSM_GetSFCErD103/1(DFC)
  DFC_DChrgTNegElecSig/1 -> DSM_GetSFCErD104/1(DFC)
  DFC_DChrgTPosElecMax/1 -> DSM_GetSFCErD105/1(DFC)
  DFC_DChrgTPosElecMin/1 -> DSM_GetSFCErD106/1(DFC)
  DFC_DChrgTPosElecSig/1 -> DSM_GetSFCErD107/1(DFC)
  DFC_CcuSelfChkErr/1 -> DSM_GetSFCErD108/1(DFC)
  DFC_ChrgOCMax/1 -> DSM_GetSFCErD119/1(DFC)
  DFC_DisChOCMin/1 -> DSM_GetSFCErD120/1(DFC)
  DFC_DisChOCMax/1 -> DSM_GetSFCErD121/1(DFC)
  DFC_SocRngLoMax/1 -> DSM_GetSFCErD122/1(DFC)
  DFC_SocRngLoMin/1 -> DSM_GetSFCErD123/1(DFC)
  DFC_SocRngHiMax/1 -> DSM_GetSFCErD124/1(DFC)
  DFC_SocRngHiMin/1 -> DSM_GetSFCErD125/1(DFC)
  DFC_InClntOverTmp/1 -> DSM_GetSFCErD126/1(DFC)
  DFC_OutClntOverTmp/1 -> DSM_GetSFCErD127/1(DFC)
  DFC_ClntDsTElecMax/1 -> DSM_GetSFCErD128/1(DFC)
  DFC_ClntDsTElecMin/1 -> DSM_GetSFCErD129/1(DFC)
  DFC_ClntDsTElecSig/1 -> DSM_GetSFCErD130/1(DFC)
  DFC_ClntUsTElecMax/1 -> DSM_GetSFCErD131/1(DFC)
  DFC_ClntUsTElecMin/1 -> DSM_GetSFCErD132/1(DFC)
  DFC_ClntUsTElecSig/1 -> DSM_GetSFCErD133/1(DFC)
  DFC_CoolPerfPlaus/1 -> DSM_GetSFCErD134/1(DFC)
  DFC_HtgPerfPlaus/1 -> DSM_GetSFCErD135/1(DFC)
  DFC_DChrgFobd/1 -> DSM_GetSFCErD136/1(DFC)
  DFC_DChrgHvOnFail/1 -> DSM_GetSFCErD137/1(DFC)
  DFC_AChgHVOnTmt/1 -> DSM_GetSFCErD138/1(DFC)
  DFC_AChgHVOffTmt/1 -> DSM_GetSFCErD139/1(DFC)
  DFC_AChgS2ClsdTmt/1 -> DSM_GetSFCErD140/1(DFC)
  DFC_DChrgStakeErr/1 -> DSM_GetSFCErD109/1(DFC)
  DFC_DChrgStkVoltErr/1 -> DSM_GetSFCErD110/1(DFC)
  DFC_DChrgStkCurrErr/1 -> DSM_GetSFCErD111/1(DFC)
  DFC_AChgPileRdyTmt/1 -> DSM_GetSFCErD112/1(DFC)
  DFC_DChrgCHMTmt/1 -> DSM_GetSFCErD113/1(DFC)
  DFC_DChrgCRMTmt/1 -> DSM_GetSFCErD114/1(DFC)
  DFC_DChrgCMLTmt/1 -> DSM_GetSFCErD115/1(DFC)
  DFC_DChrgCROTmt/1 -> DSM_GetSFCErD116/1(DFC)
  DFC_DChrgCCSTmt/1 -> DSM_GetSFCErD117/1(DFC)
  DFC_ChrgOCMin/1 -> DSM_GetSFCErD118/1(DFC)
  DFC_DChrgCSTTmt/1 -> DSM_GetSFCErD141/1(DFC)
  DFC_DChrgCSDTmt/1 -> DSM_GetSFCErD142/1(DFC)
  DFC_DChrgParaChk/1 -> DSM_GetSFCErD143/1(DFC)
  DFC_DChrgCableChk/1 -> DSM_GetSFCErD144/1(DFC)
  DFC_DChrgSLACTOut/1 -> DSM_GetSFCErD145/1(DFC)
  DFC_DChrgCnntErr/1 -> DSM_GetSFCErD146/1(DFC)
  DFC_DChrgLckErr/1 -> DSM_GetSFCErD147/1(DFC)
  DFC_AChrgCnntErr/1 -> DSM_GetSFCErD148/1(DFC)
  DFC_AChgLckTmt/1 -> DSM_GetSFCErD149/1(DFC)
  DFC_AChgRdyPndiTmt/1 -> DSM_GetSFCErD150/1(DFC)
  DFC_AChgRdyTmt/1 -> DSM_GetSFCErD151/1(DFC)
  DFC_AChgingErr/1 -> DSM_GetSFCErD152/1(DFC)
  DFC_AChgUnlckTmt/1 -> DSM_GetSFCErD153/1(DFC)
  DFC_AChgFobd/1 -> DSM_GetSFCErD154/1(DFC)
  DFC_SocValJmp/1 -> DSM_GetSFCErD155/1(DFC)
  DSM_GetSFCErD/1(y) -> Vector Concatenate/1
  DSM_GetSFCErD1/1(y) -> Vector Concatenate/2
  DSM_GetSFCErD2/1(y) -> Vector Concatenate/3
  DSM_GetSFCErD3/1(y) -> Vector Concatenate/4
  DSM_GetSFCErD4/1(y) -> Vector Concatenate/5
  DSM_GetSFCErD5/1(y) -> Vector Concatenate/6
  DSM_GetSFCErD6/1(y) -> Vector Concatenate/7
  DSM_GetSFCErD7/1(y) -> Vector Concatenate/8
  DSM_GetSFCErD8/1(y) -> Vector Concatenate/9
  DSM_GetSFCErD9/1(y) -> Vector Concatenate/10
  DSM_GetSFCErD10/1(y) -> Vector Concatenate/11
  DSM_GetSFCErD11/1(y) -> Vector Concatenate/12
  DSM_GetSFCErD12/1(y) -> Vector Concatenate/13
  DSM_GetSFCErD13/1(y) -> Vector Concatenate/14
  DSM_GetSFCErD14/1(y) -> Vector Concatenate/15
  DSM_GetSFCErD15/1(y) -> Vector Concatenate/16
  DSM_GetSFCErD16/1(y) -> Vector Concatenate/17
  DSM_GetSFCErD17/1(y) -> Vector Concatenate/18
  DSM_GetSFCErD18/1(y) -> Vector Concatenate/19
  DSM_GetSFCErD19/1(y) -> Vector Concatenate/20
  DSM_GetSFCErD20/1(y) -> Vector Concatenate/21
  DSM_GetSFCErD21/1(y) -> Vector Concatenate/22
  DSM_GetSFCErD22/1(y) -> Vector Concatenate/23
  DSM_GetSFCErD23/1(y) -> Vector Concatenate/24
  DSM_GetSFCErD24/1(y) -> Vector Concatenate/25
  DSM_GetSFCErD25/1(y) -> Vector Concatenate/26
  DSM_GetSFCErD26/1(y) -> Vector Concatenate/27
  DSM_GetSFCErD27/1(y) -> Vector Concatenate/28
  DSM_GetSFCErD28/1(y) -> Vector Concatenate/29
  DSM_GetSFCErD29/1(y) -> Vector Concatenate/30
  DSM_GetSFCErD30/1(y) -> Vector Concatenate/31
  DSM_GetSFCErD31/1(y) -> Vector Concatenate/32
  DSM_GetSFCErD32/1(y) -> Vector Concatenate/33
  DSM_GetSFCErD33/1(y) -> Vector Concatenate/34
  DSM_GetSFCErD34/1(y) -> Vector Concatenate/35
  DSM_GetSFCErD35/1(y) -> Vector Concatenate/36
  DSM_GetSFCErD36/1(y) -> Vector Concatenate/37
  DSM_GetSFCErD37/1(y) -> Vector Concatenate/38
  DSM_GetSFCErD38/1(y) -> Vector Concatenate/39
  DSM_GetSFCErD39/1(y) -> Vector Concatenate/40
  DSM_GetSFCErD40/1(y) -> Vector Concatenate/41
  DSM_GetSFCErD41/1(y) -> Vector Concatenate/42
  DSM_GetSFCErD42/1(y) -> Vector Concatenate/43
  DSM_GetSFCErD43/1(y) -> Vector Concatenate/44
  DSM_GetSFCErD44/1(y) -> Vector Concatenate/45
  DSM_GetSFCErD45/1(y) -> Vector Concatenate/46
  DSM_GetSFCErD46/1(y) -> Vector Concatenate/47
  DSM_GetSFCErD47/1(y) -> Vector Concatenate/48
  DSM_GetSFCErD48/1(y) -> Vector Concatenate/49
  DSM_GetSFCErD49/1(y) -> Vector Concatenate/50
  DSM_GetSFCErD50/1(y) -> Vector Concatenate/51
  DSM_GetSFCErD51/1(y) -> Vector Concatenate/52
  DSM_GetSFCErD52/1(y) -> Vector Concatenate/53
  DSM_GetSFCErD53/1(y) -> Vector Concatenate/54
  DSM_GetSFCErD54/1(y) -> Vector Concatenate/55
  DSM_GetSFCErD55/1(y) -> Vector Concatenate/56
  DSM_GetSFCErD56/1(y) -> Vector Concatenate/57
  DSM_GetSFCErD57/1(y) -> Vector Concatenate/58
  DSM_GetSFCErD58/1(y) -> Vector Concatenate/59
  DSM_GetSFCErD59/1(y) -> Vector Concatenate/60
  DSM_GetSFCErD60/1(y) -> Vector Concatenate/61
  DSM_GetSFCErD61/1(y) -> Vector Concatenate/62
  DSM_GetSFCErD62/1(y) -> Vector Concatenate/63
  DSM_GetSFCErD63/1(y) -> Vector Concatenate/64
  DSM_GetSFCErD64/1(y) -> Vector Concatenate/65
  DSM_GetSFCErD65/1(y) -> Vector Concatenate/66
  DSM_GetSFCErD66/1(y) -> Vector Concatenate/67
  DSM_GetSFCErD67/1(y) -> Vector Concatenate/68
  DSM_GetSFCErD68/1(y) -> Vector Concatenate/69
  DSM_GetSFCErD69/1(y) -> Vector Concatenate/70
  DSM_GetSFCErD70/1(y) -> Vector Concatenate/71
  DSM_GetSFCErD71/1(y) -> Vector Concatenate/72
  DSM_GetSFCErD72/1(y) -> Vector Concatenate/73
  DSM_GetSFCErD73/1(y) -> Vector Concatenate/74
  DSM_GetSFCErD74/1(y) -> Vector Concatenate/75
  DSM_GetSFCErD75/1(y) -> Vector Concatenate/76
  DSM_GetSFCErD76/1(y) -> Vector Concatenate/77
  DSM_GetSFCErD77/1(y) -> Vector Concatenate/78
  DSM_GetSFCErD78/1(y) -> Vector Concatenate/79
  DSM_GetSFCErD79/1(y) -> Vector Concatenate/80
  DSM_GetSFCErD80/1(y) -> Vector Concatenate/81
  DSM_GetSFCErD81/1(y) -> Vector Concatenate/82
  DSM_GetSFCErD82/1(y) -> Vector Concatenate/83
  DSM_GetSFCErD83/1(y) -> Vector Concatenate/84
  DSM_GetSFCErD84/1(y) -> Vector Concatenate/85
  DSM_GetSFCErD85/1(y) -> Vector Concatenate/86
  DSM_GetSFCErD86/1(y) -> Vector Concatenate/87
  DSM_GetSFCErD87/1(y) -> Vector Concatenate/88
  DSM_GetSFCErD88/1(y) -> Vector Concatenate/89
  DSM_GetSFCErD89/1(y) -> Vector Concatenate/90
  DSM_GetSFCErD90/1(y) -> Vector Concatenate/91
  DSM_GetSFCErD91/1(y) -> Vector Concatenate/92
  DSM_GetSFCErD92/1(y) -> Vector Concatenate/93
  DSM_GetSFCErD93/1(y) -> Vector Concatenate/94
  DSM_GetSFCErD94/1(y) -> Vector Concatenate/95
  DSM_GetSFCErD95/1(y) -> Vector Concatenate/96
  DSM_GetSFCErD96/1(y) -> Vector Concatenate/97
  DSM_GetSFCErD97/1(y) -> Vector Concatenate/98
  DSM_GetSFCErD98/1(y) -> Vector Concatenate/99
  DSM_GetSFCErD99/1(y) -> Vector Concatenate/100
  DSM_GetSFCErD100/1(y) -> Vector Concatenate/101
  DSM_GetSFCErD101/1(y) -> Vector Concatenate/102
  DSM_GetSFCErD102/1(y) -> Vector Concatenate/103
  DSM_GetSFCErD103/1(y) -> Vector Concatenate/104
  DSM_GetSFCErD104/1(y) -> Vector Concatenate/105
  DSM_GetSFCErD105/1(y) -> Vector Concatenate/106
  DSM_GetSFCErD106/1(y) -> Vector Concatenate/107
  DSM_GetSFCErD107/1(y) -> Vector Concatenate/108
  DSM_GetSFCErD108/1(y) -> Vector Concatenate/109
  DSM_GetSFCErD118/1(y) -> Vector Concatenate/110
  DSM_GetSFCErD119/1(y) -> Vector Concatenate/111
  DSM_GetSFCErD120/1(y) -> Vector Concatenate/112
  DSM_GetSFCErD121/1(y) -> Vector Concatenate/113
  DSM_GetSFCErD122/1(y) -> Vector Concatenate/114
  DSM_GetSFCErD123/1(y) -> Vector Concatenate/115
  DSM_GetSFCErD124/1(y) -> Vector Concatenate/116
  DSM_GetSFCErD125/1(y) -> Vector Concatenate/117
  DSM_GetSFCErD126/1(y) -> Vector Concatenate/118
  DSM_GetSFCErD127/1(y) -> Vector Concatenate/119
  DSM_GetSFCErD128/1(y) -> Vector Concatenate/120
  DSM_GetSFCErD129/1(y) -> Vector Concatenate/121
  DSM_GetSFCErD130/1(y) -> Vector Concatenate/122
  DSM_GetSFCErD131/1(y) -> Vector Concatenate/123
  DSM_GetSFCErD132/1(y) -> Vector Concatenate/124
  DSM_GetSFCErD133/1(y) -> Vector Concatenate/125
  DSM_GetSFCErD134/1(y) -> Vector Concatenate/126
  DSM_GetSFCErD135/1(y) -> Vector Concatenate/127
  DSM_GetSFCErD136/1(y) -> Vector Concatenate/128
  DSM_GetSFCErD137/1(y) -> Vector Concatenate/129
  DSM_GetSFCErD138/1(y) -> Vector Concatenate/130
  DSM_GetSFCErD139/1(y) -> Vector Concatenate/131
  DSM_GetSFCErD140/1(y) -> Vector Concatenate/132
  DSM_GetSFCErD109/1(y) -> Vector Concatenate/133
  DSM_GetSFCErD110/1(y) -> Vector Concatenate/134
  DSM_GetSFCErD111/1(y) -> Vector Concatenate/135
  DSM_GetSFCErD112/1(y) -> Vector Concatenate/136
  DSM_GetSFCErD113/1(y) -> Vector Concatenate/137
  DSM_GetSFCErD114/1(y) -> Vector Concatenate/138
  DSM_GetSFCErD115/1(y) -> Vector Concatenate/139
  DSM_GetSFCErD116/1(y) -> Vector Concatenate/140
  DSM_GetSFCErD117/1(y) -> Vector Concatenate/141
  DSM_GetSFCErD141/1(y) -> Vector Concatenate/142
  DSM_GetSFCErD142/1(y) -> Vector Concatenate/143
  DSM_GetSFCErD143/1(y) -> Vector Concatenate/144
  DSM_GetSFCErD144/1(y) -> Vector Concatenate/145
  DSM_GetSFCErD145/1(y) -> Vector Concatenate/146
  DSM_GetSFCErD146/1(y) -> Vector Concatenate/147
  DSM_GetSFCErD147/1(y) -> Vector Concatenate/148
  DSM_GetSFCErD148/1(y) -> Vector Concatenate/149
  DSM_GetSFCErD149/1(y) -> Vector Concatenate/150
  DSM_GetSFCErD150/1(y) -> Vector Concatenate/151
  DSM_GetSFCErD151/1(y) -> Vector Concatenate/152
  DSM_GetSFCErD152/1(y) -> Vector Concatenate/153
  DSM_GetSFCErD153/1(y) -> Vector Concatenate/154
  DSM_GetSFCErD154/1(y) -> Vector Concatenate/155
  DSM_GetSFCErD155/1(y) -> Vector Concatenate/156
  Vector Concatenate/1 -> FaultStatus/1

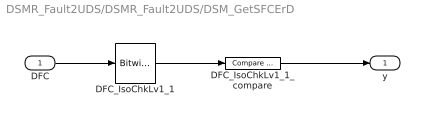
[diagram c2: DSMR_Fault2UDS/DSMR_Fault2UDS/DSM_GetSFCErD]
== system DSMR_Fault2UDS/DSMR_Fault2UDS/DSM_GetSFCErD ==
  DFC : Inport  OutDataTypeStr=uint8
  DFC_IsoChkLv1_1 : simulink/Logic and Bit Operations/Bitwise Operator  logicop=AND  UseBitMask=on  BitMask=bin2dec('00011000')  BitMaskRealWorld=Stored Integer
  DFC_IsoChkLv1_1_compare : simulink/Logic and Bit Operations/Compare To Constant  relop===  const=24  OutDataTypeStr=boolean
  y : Outport
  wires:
  DFC_IsoChkLv1_1_compare/1 -> y/1
  DFC/1 -> DFC_IsoChkLv1_1/1
  DFC_IsoChkLv1_1/1 -> DFC_IsoChkLv1_1_compare/1

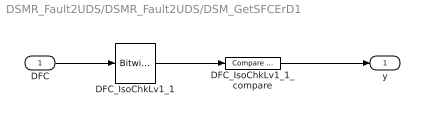
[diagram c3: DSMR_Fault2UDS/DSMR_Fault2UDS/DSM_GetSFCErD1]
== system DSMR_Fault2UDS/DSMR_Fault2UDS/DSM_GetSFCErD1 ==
  DFC : Inport  OutDataTypeStr=uint8
  DFC_IsoChkLv1_1 : simulink/Logic and Bit Operations/Bitwise Operator  logicop=AND  UseBitMask=on  BitMask=bin2dec('00011000')  BitMaskRealWorld=Stored Integer
  DFC_IsoChkLv1_1_compare : simulink/Logic and Bit Operations/Compare To Constant  relop===  const=24  OutDataTypeStr=boolean
  y : Outport
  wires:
  DFC_IsoChkLv1_1_compare/1 -> y/1
  DFC/1 -> DFC_IsoChkLv1_1/1
  DFC_IsoChkLv1_1/1 -> DFC_IsoChkLv1_1_compare/1

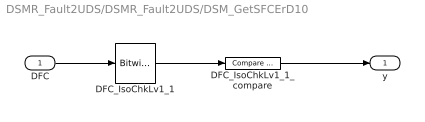
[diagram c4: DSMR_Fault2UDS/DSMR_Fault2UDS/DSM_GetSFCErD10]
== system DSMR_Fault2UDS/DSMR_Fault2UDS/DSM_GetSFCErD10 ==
  DFC : Inport  OutDataTypeStr=uint8
  DFC_IsoChkLv1_1 : simulink/Logic and Bit Operations/Bitwise Operator  logicop=AND  UseBitMask=on  BitMask=bin2dec('00011000')  BitMaskRealWorld=Stored Integer
  DFC_IsoChkLv1_1_compare : simulink/Logic and Bit Operations/Compare To Constant  relop===  const=24  OutDataTypeStr=boolean
  y : Outport
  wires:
  DFC_IsoChkLv1_1_compare/1 -> y/1
  DFC/1 -> DFC_IsoChkLv1_1/1
  DFC_IsoChkLv1_1/1 -> DFC_IsoChkLv1_1_compare/1

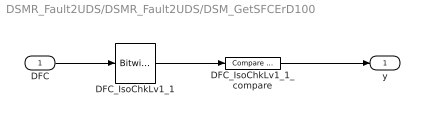
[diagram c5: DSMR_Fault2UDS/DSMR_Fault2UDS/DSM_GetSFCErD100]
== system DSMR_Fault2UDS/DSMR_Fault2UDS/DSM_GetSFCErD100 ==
  DFC : Inport  OutDataTypeStr=uint8
  DFC_IsoChkLv1_1 : simulink/Logic and Bit Operations/Bitwise Operator  logicop=AND  UseBitMask=on  BitMask=bin2dec('00011000')  BitMaskRealWorld=Stored Integer
  DFC_IsoChkLv1_1_compare : simulink/Logic and Bit Operations/Compare To Constant  relop===  const=24  OutDataTypeStr=boolean
  y : Outport
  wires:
  DFC_IsoChkLv1_1_compare/1 -> y/1
  DFC/1 -> DFC_IsoChkLv1_1/1
  DFC_IsoChkLv1_1/1 -> DFC_IsoChkLv1_1_compare/1

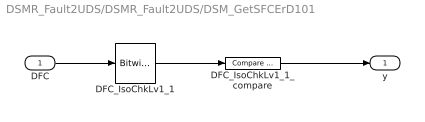
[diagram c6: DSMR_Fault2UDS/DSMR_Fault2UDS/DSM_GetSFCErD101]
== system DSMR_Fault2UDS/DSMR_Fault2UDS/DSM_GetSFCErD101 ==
  DFC : Inport  OutDataTypeStr=uint8
  DFC_IsoChkLv1_1 : simulink/Logic and Bit Operations/Bitwise Operator  logicop=AND  UseBitMask=on  BitMask=bin2dec('00011000')  BitMaskRealWorld=Stored Integer
  DFC_IsoChkLv1_1_compare : simulink/Logic and Bit Operations/Compare To Constant  relop===  const=24  OutDataTypeStr=boolean
  y : Outport
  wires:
  DFC_IsoChkLv1_1_compare/1 -> y/1
  DFC/1 -> DFC_IsoChkLv1_1/1
  DFC_IsoChkLv1_1/1 -> DFC_IsoChkLv1_1_compare/1

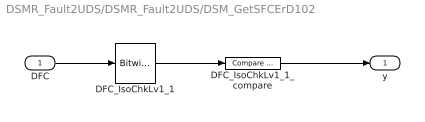
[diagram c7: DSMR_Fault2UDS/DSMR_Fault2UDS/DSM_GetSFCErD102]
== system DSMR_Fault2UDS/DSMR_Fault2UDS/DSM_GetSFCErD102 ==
  DFC : Inport  OutDataTypeStr=uint8
  DFC_IsoChkLv1_1 : simulink/Logic and Bit Operations/Bitwise Operator  logicop=AND  UseBitMask=on  BitMask=bin2dec('00011000')  BitMaskRealWorld=Stored Integer
  DFC_IsoChkLv1_1_compare : simulink/Logic and Bit Operations/Compare To Constant  relop===  const=24  OutDataTypeStr=boolean
  y : Outport
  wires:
  DFC_IsoChkLv1_1_compare/1 -> y/1
  DFC/1 -> DFC_IsoChkLv1_1/1
  DFC_IsoChkLv1_1/1 -> DFC_IsoChkLv1_1_compare/1

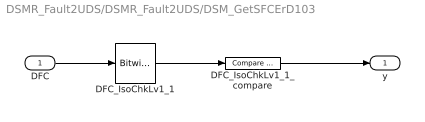
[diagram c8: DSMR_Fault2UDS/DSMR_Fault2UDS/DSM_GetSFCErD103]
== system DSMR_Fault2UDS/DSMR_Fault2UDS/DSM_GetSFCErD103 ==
  DFC : Inport  OutDataTypeStr=uint8
  DFC_IsoChkLv1_1 : simulink/Logic and Bit Operations/Bitwise Operator  logicop=AND  UseBitMask=on  BitMask=bin2dec('00011000')  BitMaskRealWorld=Stored Integer
  DFC_IsoChkLv1_1_compare : simulink/Logic and Bit Operations/Compare To Constant  relop===  const=24  OutDataTypeStr=boolean
  y : Outport
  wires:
  DFC_IsoChkLv1_1_compare/1 -> y/1
  DFC/1 -> DFC_IsoChkLv1_1/1
  DFC_IsoChkLv1_1/1 -> DFC_IsoChkLv1_1_compare/1

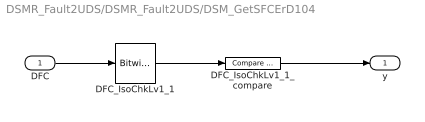
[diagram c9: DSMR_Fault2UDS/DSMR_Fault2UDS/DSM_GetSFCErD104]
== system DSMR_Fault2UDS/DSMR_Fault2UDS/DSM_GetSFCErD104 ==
  DFC : Inport  OutDataTypeStr=uint8
  DFC_IsoChkLv1_1 : simulink/Logic and Bit Operations/Bitwise Operator  logicop=AND  UseBitMask=on  BitMask=bin2dec('00011000')  BitMaskRealWorld=Stored Integer
  DFC_IsoChkLv1_1_compare : simulink/Logic and Bit Operations/Compare To Constant  relop===  const=24  OutDataTypeStr=boolean
  y : Outport
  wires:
  DFC_IsoChkLv1_1_compare/1 -> y/1
  DFC/1 -> DFC_IsoChkLv1_1/1
  DFC_IsoChkLv1_1/1 -> DFC_IsoChkLv1_1_compare/1

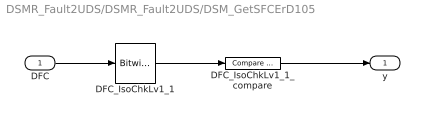
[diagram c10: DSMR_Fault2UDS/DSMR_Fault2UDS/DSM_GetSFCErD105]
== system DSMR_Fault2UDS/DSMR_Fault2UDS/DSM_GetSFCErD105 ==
  DFC : Inport  OutDataTypeStr=uint8
  DFC_IsoChkLv1_1 : simulink/Logic and Bit Operations/Bitwise Operator  logicop=AND  UseBitMask=on  BitMask=bin2dec('00011000')  BitMaskRealWorld=Stored Integer
  DFC_IsoChkLv1_1_compare : simulink/Logic and Bit Operations/Compare To Constant  relop===  const=24  OutDataTypeStr=boolean
  y : Outport
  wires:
  DFC_IsoChkLv1_1_compare/1 -> y/1
  DFC/1 -> DFC_IsoChkLv1_1/1
  DFC_IsoChkLv1_1/1 -> DFC_IsoChkLv1_1_compare/1

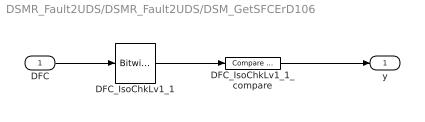
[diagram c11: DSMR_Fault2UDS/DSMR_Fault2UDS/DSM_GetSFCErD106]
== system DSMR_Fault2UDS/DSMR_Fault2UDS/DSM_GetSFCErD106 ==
  DFC : Inport  OutDataTypeStr=uint8
  DFC_IsoChkLv1_1 : simulink/Logic and Bit Operations/Bitwise Operator  logicop=AND  UseBitMask=on  BitMask=bin2dec('00011000')  BitMaskRealWorld=Stored Integer
  DFC_IsoChkLv1_1_compare : simulink/Logic and Bit Operations/Compare To Constant  relop===  const=24  OutDataTypeStr=boolean
  y : Outport
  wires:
  DFC_IsoChkLv1_1_compare/1 -> y/1
  DFC/1 -> DFC_IsoChkLv1_1/1
  DFC_IsoChkLv1_1/1 -> DFC_IsoChkLv1_1_compare/1

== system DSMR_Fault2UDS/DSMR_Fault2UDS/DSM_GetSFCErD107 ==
  DFC : Inport  OutDataTypeStr=uint8
  DFC_IsoChkLv1_1 : simulink/Logic and Bit Operations/Bitwise Operator  logicop=AND  UseBitMask=on  BitMask=bin2dec('00011000')  BitMaskRealWorld=Stored Integer
  DFC_IsoChkLv1_1_compare : simulink/Logic and Bit Operations/Compare To Constant  relop===  const=24  OutDataTypeStr=boolean
  y : Outport
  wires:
  DFC_IsoChkLv1_1_compare/1 -> y/1
  DFC/1 -> DFC_IsoChkLv1_1/1
  DFC_IsoChkLv1_1/1 -> DFC_IsoChkLv1_1_compare/1

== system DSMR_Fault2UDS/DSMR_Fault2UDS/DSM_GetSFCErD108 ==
  DFC : Inport  OutDataTypeStr=uint8
  DFC_IsoChkLv1_1 : simulink/Logic and Bit Operations/Bitwise Operator  logicop=AND  UseBitMask=on  BitMask=bin2dec('00011000')  BitMaskRealWorld=Stored Integer
  DFC_IsoChkLv1_1_compare : simulink/Logic and Bit Operations/Compare To Constant  relop===  const=24  OutDataTypeStr=boolean
  y : Outport
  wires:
  DFC_IsoChkLv1_1_compare/1 -> y/1
  DFC/1 -> DFC_IsoChkLv1_1/1
  DFC_IsoChkLv1_1/1 -> DFC_IsoChkLv1_1_compare/1

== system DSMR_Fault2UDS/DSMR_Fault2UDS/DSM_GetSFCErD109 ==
  DFC : Inport  OutDataTypeStr=uint8
  DFC_IsoChkLv1_1 : simulink/Logic and Bit Operations/Bitwise Operator  logicop=AND  UseBitMask=on  BitMask=bin2dec('00011000')  BitMaskRealWorld=Stored Integer
  DFC_IsoChkLv1_1_compare : simulink/Logic and Bit Operations/Compare To Constant  relop===  const=24  OutDataTypeStr=boolean
  y : Outport
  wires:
  DFC_IsoChkLv1_1_compare/1 -> y/1
  DFC/1 -> DFC_IsoChkLv1_1/1
  DFC_IsoChkLv1_1/1 -> DFC_IsoChkLv1_1_compare/1

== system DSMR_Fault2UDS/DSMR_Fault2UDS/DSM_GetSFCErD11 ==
  DFC : Inport  OutDataTypeStr=uint8
  DFC_IsoChkLv1_1 : simulink/Logic and Bit Operations/Bitwise Operator  logicop=AND  UseBitMask=on  BitMask=bin2dec('00011000')  BitMaskRealWorld=Stored Integer
  DFC_IsoChkLv1_1_compare : simulink/Logic and Bit Operations/Compare To Constant  relop===  const=24  OutDataTypeStr=boolean
  y : Outport
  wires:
  DFC_IsoChkLv1_1_compare/1 -> y/1
  DFC/1 -> DFC_IsoChkLv1_1/1
  DFC_IsoChkLv1_1/1 -> DFC_IsoChkLv1_1_compare/1

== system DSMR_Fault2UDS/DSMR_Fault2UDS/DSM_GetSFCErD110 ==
  DFC : Inport  OutDataTypeStr=uint8
  DFC_IsoChkLv1_1 : simulink/Logic and Bit Operations/Bitwise Operator  logicop=AND  UseBitMask=on  BitMask=bin2dec('00011000')  BitMaskRealWorld=Stored Integer
  DFC_IsoChkLv1_1_compare : simulink/Logic and Bit Operations/Compare To Constant  relop===  const=24  OutDataTypeStr=boolean
  y : Outport
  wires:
  DFC_IsoChkLv1_1_compare/1 -> y/1
  DFC/1 -> DFC_IsoChkLv1_1/1
  DFC_IsoChkLv1_1/1 -> DFC_IsoChkLv1_1_compare/1

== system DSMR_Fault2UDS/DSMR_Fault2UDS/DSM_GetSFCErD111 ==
  DFC : Inport  OutDataTypeStr=uint8
  DFC_IsoChkLv1_1 : simulink/Logic and Bit Operations/Bitwise Operator  logicop=AND  UseBitMask=on  BitMask=bin2dec('00011000')  BitMaskRealWorld=Stored Integer
  DFC_IsoChkLv1_1_compare : simulink/Logic and Bit Operations/Compare To Constant  relop===  const=24  OutDataTypeStr=boolean
  y : Outport
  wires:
  DFC_IsoChkLv1_1_compare/1 -> y/1
  DFC/1 -> DFC_IsoChkLv1_1/1
  DFC_IsoChkLv1_1/1 -> DFC_IsoChkLv1_1_compare/1

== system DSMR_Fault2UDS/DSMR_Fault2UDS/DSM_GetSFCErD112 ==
  DFC : Inport  OutDataTypeStr=uint8
  DFC_IsoChkLv1_1 : simulink/Logic and Bit Operations/Bitwise Operator  logicop=AND  UseBitMask=on  BitMask=bin2dec('00011000')  BitMaskRealWorld=Stored Integer
  DFC_IsoChkLv1_1_compare : simulink/Logic and Bit Operations/Compare To Constant  relop===  const=24  OutDataTypeStr=boolean
  y : Outport
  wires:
  DFC_IsoChkLv1_1_compare/1 -> y/1
  DFC/1 -> DFC_IsoChkLv1_1/1
  DFC_IsoChkLv1_1/1 -> DFC_IsoChkLv1_1_compare/1

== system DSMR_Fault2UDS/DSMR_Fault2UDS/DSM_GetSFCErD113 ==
  DFC : Inport  OutDataTypeStr=uint8
  DFC_IsoChkLv1_1 : simulink/Logic and Bit Operations/Bitwise Operator  logicop=AND  UseBitMask=on  BitMask=bin2dec('00011000')  BitMaskRealWorld=Stored Integer
  DFC_IsoChkLv1_1_compare : simulink/Logic and Bit Operations/Compare To Constant  relop===  const=24  OutDataTypeStr=boolean
  y : Outport
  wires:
  DFC_IsoChkLv1_1_compare/1 -> y/1
  DFC/1 -> DFC_IsoChkLv1_1/1
  DFC_IsoChkLv1_1/1 -> DFC_IsoChkLv1_1_compare/1

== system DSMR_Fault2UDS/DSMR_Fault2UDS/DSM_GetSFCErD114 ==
  DFC : Inport  OutDataTypeStr=uint8
  DFC_IsoChkLv1_1 : simulink/Logic and Bit Operations/Bitwise Operator  logicop=AND  UseBitMask=on  BitMask=bin2dec('00011000')  BitMaskRealWorld=Stored Integer
  DFC_IsoChkLv1_1_compare : simulink/Logic and Bit Operations/Compare To Constant  relop===  const=24  OutDataTypeStr=boolean
  y : Outport
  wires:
  DFC_IsoChkLv1_1_compare/1 -> y/1
  DFC/1 -> DFC_IsoChkLv1_1/1
  DFC_IsoChkLv1_1/1 -> DFC_IsoChkLv1_1_compare/1

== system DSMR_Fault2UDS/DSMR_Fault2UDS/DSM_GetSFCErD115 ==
  DFC : Inport  OutDataTypeStr=uint8
  DFC_IsoChkLv1_1 : simulink/Logic and Bit Operations/Bitwise Operator  logicop=AND  UseBitMask=on  BitMask=bin2dec('00011000')  BitMaskRealWorld=Stored Integer
  DFC_IsoChkLv1_1_compare : simulink/Logic and Bit Operations/Compare To Constant  relop===  const=24  OutDataTypeStr=boolean
  y : Outport
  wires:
  DFC_IsoChkLv1_1_compare/1 -> y/1
  DFC/1 -> DFC_IsoChkLv1_1/1
  DFC_IsoChkLv1_1/1 -> DFC_IsoChkLv1_1_compare/1

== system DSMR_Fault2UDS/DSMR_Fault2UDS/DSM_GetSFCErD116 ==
  DFC : Inport  OutDataTypeStr=uint8
  DFC_IsoChkLv1_1 : simulink/Logic and Bit Operations/Bitwise Operator  logicop=AND  UseBitMask=on  BitMask=bin2dec('00011000')  BitMaskRealWorld=Stored Integer
  DFC_IsoChkLv1_1_compare : simulink/Logic and Bit Operations/Compare To Constant  relop===  const=24  OutDataTypeStr=boolean
  y : Outport
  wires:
  DFC_IsoChkLv1_1_compare/1 -> y/1
  DFC/1 -> DFC_IsoChkLv1_1/1
  DFC_IsoChkLv1_1/1 -> DFC_IsoChkLv1_1_compare/1

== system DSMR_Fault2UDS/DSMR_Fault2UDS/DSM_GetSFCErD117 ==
  DFC : Inport  OutDataTypeStr=uint8
  DFC_IsoChkLv1_1 : simulink/Logic and Bit Operations/Bitwise Operator  logicop=AND  UseBitMask=on  BitMask=bin2dec('00011000')  BitMaskRealWorld=Stored Integer
  DFC_IsoChkLv1_1_compare : simulink/Logic and Bit Operations/Compare To Constant  relop===  const=24  OutDataTypeStr=boolean
  y : Outport
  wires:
  DFC_IsoChkLv1_1_compare/1 -> y/1
  DFC/1 -> DFC_IsoChkLv1_1/1
  DFC_IsoChkLv1_1/1 -> DFC_IsoChkLv1_1_compare/1
